ORGANIZATION_BLOCK MAIN:OB1
TITLE= Avviatore Stella-Triangolo per M.A.T.
// Simulatore:02
// Versione: 1.0
// Data: 03/03/2002
// Il programma consente di effettuare l'avviamento Stella-Triangolo
// di un motore asincrono trifase.
// Il motore viene comandato da tre contattori KM1, KM2, KM3; in
// particolare KM1 consente di alimentare il motore (linea),
// KM2 effetua il temporaneo collegamento a stella e KM3 consente,
// dopo la fase di avviamento, il definitivo collegamento a triangolo.
// Per motivi di sicurezza si è scelto di disattivare, in caso di
// intervento del relè termico FR, le uscite più critiche (Q0.0, Q0.1,
// Q0.2), quelle cioè che comandano i contattori, non solo via
// hardware, ma anche via software riportando su un ingresso un
// contatto ausiliario (NO) di KM1 per testare lo stato effetivo
// del contattore.
// Il motore viene avviato dal pulsante (NO) SB2 e può essere
// arrestato in qualsiasi momento dal pulsante (NC) SB1.
// Dopo un eventuale intervento del relè termico FR e il suo
// ripristino, è necessario riavviare il motore mediante il pulsante
// di marcia SB2.
// Il programma prevede il controllo dell'effetiva chiusura del
// contattore KM3 (triangolo); se l'effettiva chiusura non avviene nel
// tempo previsto (T33) il PLC disattiva automaticamente tutti i
// contattori.
// I contattori KM2 e KM3 non devono poter essere inseriti
// conteporaneamente (corto circuito sulla linea di potenza), è
// quindi necessario prevedere un interblocco elettrico harware;
// questo interblocco viene però replicato dal programma via
// software.
// Le segnalazioni sono affidate a tre lampade:
// - HL1 motore fermo
// - HL2 marcia a stella
// - HL3 marcia a triangolo.
//

BEGIN
NETWORK 1 //Imposta (SET) Bit SCR
//
LD I0.0
AN T33
S S0.0 1

NETWORK 2 //Imposta (RESET) bit SCR
//
LDN I0.0
O T33
LD I0.4
A I0.3
OLD
R S0.0 1

NETWORK 3 //Inizio segmento SCR
//
LSCR S0.0

NETWORK 4
LD Q0.0
A I0.2
O I0.1
= Q0.0

NETWORK 5 //Gestione contattore di linea
//
LD Q0.0
TON T32 +50

NETWORK 6 //Gestione contattore stella
//
LD Q0.1
A I0.4
O I0.1
AN T32
AN I0.3
= Q0.1

NETWORK 7 //Gestione contattore triangolo
//
LD T32
A Q0.0
AN I0.4
= Q0.2

NETWORK 8 //Test su chiusura effetiva contattore Triangolo
//
LD Q0.2
AN I0.3
TON T33 +5

NETWORK 9 //Fine segmento SCR
//
SCRE

NETWORK 10 //Segnalazione motore fermo
//
LDN Q0.0
= Q0.3

NETWORK 11 //Segnalazione marcia stella
//
LD Q0.1
= Q0.4

NETWORK 12 //Segbalazione marcia triangolo
//
LD Q0.2
= Q0.5

END_ORGANIZATION_BLOCK

